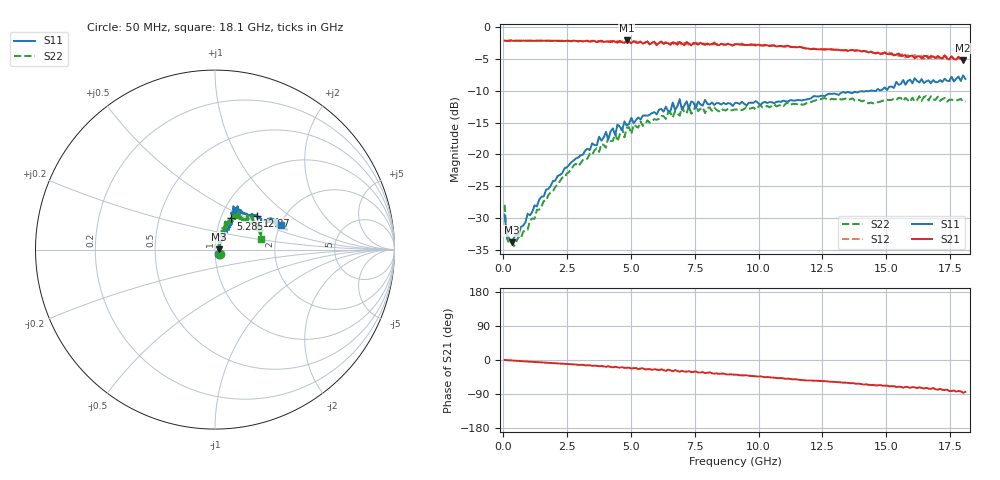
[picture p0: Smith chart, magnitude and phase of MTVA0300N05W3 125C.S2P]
! Network Analyzer HP8720D.06.14 Serial No. US36140669
!  7 Jul 2005  09:34:00
! Frequency  S11  S21  S12  S22
# HZ  S  DB R 50
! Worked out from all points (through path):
!   201 points, 50 MHz to 18.1 GHz, reference 50 ohm
!   highest |S21| = -2.07 dB at 4.833 GHz (marker M1); lowest = -5.1 dB at 18.01 GHz (marker M2)
!   group delay of S21, straight-line fit = 12.8 ps
!   lowest |S11| = -33.8 dB at 320.8 MHz (marker M3), VSWR 1.04, Z = 52.1 + j0.19 ohm
!   |S11| at or under -10 dB: start of sweep to 14.36 GHz; 14.52289 GHz to 14.58963 GHz (66.74 MHz wide, 0.458 % of centre)
!   |S22| runs from -34.4 to -10.8 dB; largest |S21 - S12| = 0.048
!   S11 on the Smith chart (normalised r, x): 50 MHz: 1.05, -0.05; 5.285 GHz: 1.12, +0.40; 12.87 GHz: 1.47, +0.60; 18.1 GHz: 2.02, +0.65
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5e7  -29.46 -43.8  -2.10 0.1  -2.09 0.3  -27.92 -40.6
1.4025e8  -32.60 -22.9  -2.16 -0.4  -2.14 -0.5  -33.20 -23.5
3.2075e8  -33.80 5.1  -2.08 -1.1  -2.10 -1.0  -33.81 2.4
1.94525e9  -24.17 54.0  -2.14 -8.3  -2.13 -8.2  -25.82 61.9
3.1185e9  -20.04 58.4  -2.20 -12.7  -2.23 -13.2  -20.87 69.3
4.021e9  -16.46 60.5  -2.22 -17.9  -2.24 -16.7  -18.93 66.6
4.11125e9  -17.67 60.9  -2.20 -16.5  -2.30 -18.1  -17.21 66.7
4.83325e9  -15.49 65.2  -2.07 -20.6  -2.35 -21.3  -15.85 60.9
5.2845e9  -14.18 62.7  -2.42 -24.2  -2.47 -23.2  -15.78 60.6
6.09675e9  -12.97 60.0  -2.46 -26.8  -2.33 -26.4  -14.39 61.3
6.7285e9  -13.00 66.4  -2.48 -26.6  -2.81 -27.5  -13.18 56.2
6.909e9  -11.30 62.6  -2.30 -30.8  -2.38 -28.5  -13.90 56.9
6.99925e9  -13.00 62.7  -2.56 -28.6  -2.78 -31.0  -12.50 57.0
7.36025e9  -11.67 57.2  -2.85 -31.9  -2.43 -30.8  -13.59 60.3
7.54075e9  -12.74 60.2  -2.57 -30.0  -2.44 -33.5  -12.09 58.6
7.90175e9  -11.42 61.5  -2.76 -34.5  -2.59 -32.4  -13.49 54.9
9.075e9  -11.89 59.8  -2.67 -38.8  -2.64 -38.8  -12.90 49.0
1.21435e10  -10.85 43.6  -3.40 -54.2  -3.33 -54.3  -11.61 45.4
1.28655e10  -10.48 38.5  -3.49 -57.3  -3.47 -57.6  -11.24 41.4
1.512175e10  -9.35 26.7  -4.24 -69.8  -3.98 -69.4  -11.45 33.2
1.800975e10  -7.57 15.6  -5.13 -86.3  -4.86 -86.5  -11.70 17.3
1.81e10  -8.12 20.3  -5.01 -84.0  -5.30 -83.8  -11.58 13.1
